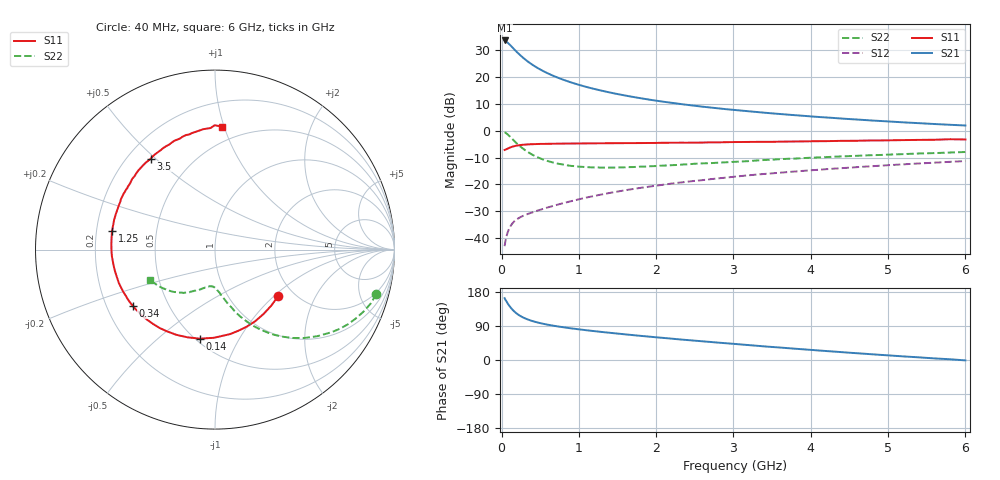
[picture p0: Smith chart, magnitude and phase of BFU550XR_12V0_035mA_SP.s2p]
! Filename:  P:\Prog\Test\Noise\ATS_data\Testdata_Net\03 Spar\BFU550XR_APG2013_45_C05_12p0V_035mA_SP_CM01_D.s2p
! Date/Time: Tue 06/Aug/2013 14:38:19
! BFU550XR_APG2013_45_C05_12p0V_25to35mA_SP_CM01_Bias2_R.s2p
! MDIF S-parameter v. bias file
! BFU550XR_APG2013_45_C05_12p0V_25to35mA_SP_CM01
! Date/time Mon Aug 05 17:40:26 2013
! VAR V_out= 12.0010
! VAR I_out= 35.0000
! VAR V_in= 0.7482
! VAR I_in= 0.3430
! Device data file deembeded for feedlines and parallel
! Original file: \03 Spar\BFU550XR_APG2013_45_C05_12p0V_035mA_SP_CM01_R.s2p
! Feed-files: PR006V01_02082013_Feed1.s2p, PR006V01_02082013_Feed2.s2p
! Parallel-file: PR006V01_02082013_Par.s2p
# MHz S MA R 50
!  Freq-MHz  S11-mag  S11-arg  S21-mag  S21-arg  S12-mag  S12-arg  S22-mag  S22-arg
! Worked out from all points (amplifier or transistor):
!   98 points, 40 MHz to 6 GHz, reference 50 ohm
!   highest |S21| = 33.7 dB at 40 MHz (marker M1)
!   |S21| within 3 dB of that: start of sweep to 154.2 MHz
!   unconditionally stable (mu >= 1): 1.302 GHz to 3.116 GHz
!   at 300 MHz: K = 0.54, MSG = 29.1 dB, |S12| = -31.5 dB
!   at 1.6 GHz: K = 1.02, MAG = 16.8 dB, |S12| = -22.2 dB
!   at 6 GHz: K = 0.87, MSG = 6.6 dB, |S12| = -11.3 dB
!   S11 on the Smith chart (normalised r, x): 40 MHz: 1.66, -1.06; 140 MHz: 0.52, -0.70; 340 MHz: 0.31, -0.28; 1.25 GHz: 0.27, +0.08; 3.5 GHz: 0.29, +0.48; 6 GHz: 0.38, +0.98
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40  0.4369 -36.5  48.2 163.2  0.007024 75.9  0.9322 -15.4
50  0.4425 -44.9  47.04 158.9  0.008639 74.5  0.9179 -19.1
80  0.4644 -67.6  43.74 149.3  0.01275 67.5  0.8494 -29.3
90  0.4705 -74.0  42.36 146.1  0.01394 65.6  0.8234 -32.4
120  0.4914 -90.7  38.46 137.9  0.01694 60.6  0.7465 -40.3
140  0.5036 -99.7  35.91 133.2  0.01861 58.2  0.6983 -44.9
180  0.5213 -114.3  31.21 125.4  0.02131 54.5  0.6124 -52.3
220  0.5348 -125.2  27.43 119.2  0.02331 52.5  0.5419 -58.0
280  0.5475 -137.3  22.9 112.2  0.02584 51.1  0.4609 -64.4
340  0.5551 -145.9  19.52 106.9  0.02801 51.1  0.402 -69.0
400  0.5597 -152.7  16.97 102.7  0.02996 51.7  0.3558 -72.6
460  0.5642 -157.7  14.97 99.4  0.03215 52.5  0.3228 -75.3
650  0.5711 -169.7  10.86 91.2  0.03891 55.6  0.2589 -81.9
850  0.5763 -178.1  8.411 84.9  0.04651 58.1  0.226 -86.8
1050  0.5787 175.4  6.844 79.7  0.05457 59.9  0.2116 -90.3
1250  0.5825 169.8  5.774 75.1  0.06284 60.7  0.2062 -94.0
2050  0.5943 152.0  3.543 59.0  0.09646 60.1  0.2223 -105.6
3100  0.6154 132.1  2.374 41.0  0.1428 55.2  0.2662 -118.8
3500  0.62 125.2  2.105 34.4  0.1603 52.3  0.2883 -123.9
4100  0.6374 115.2  1.804 25.1  0.187 48.2  0.3172 -131.2
5200  0.668 97.9  1.43 9.5  0.2359 39.5  0.3662 -144.8
6000  0.6862 86.7  1.25 -1.0  0.2715 32.4  0.4007 -155.0
